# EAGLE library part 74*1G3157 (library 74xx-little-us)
Single-Pole, Double-Throw Analog Switch Source: http://focus.ti.com/lit/ds/symlink/sn74lvc1g3157.pdf
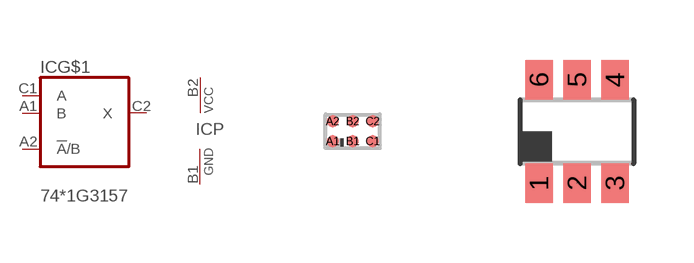
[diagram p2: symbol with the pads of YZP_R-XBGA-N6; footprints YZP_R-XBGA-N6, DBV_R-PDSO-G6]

Designator prefix IC; gates G$1=743157 P=PWRN-1

## 741G3157ZYPR  [YZP_R-XBGA-N6]
A1  G$1:B
A2  G$1:!A!/B  in
B1  P:GND  pwr
B2  P:VCC  pwr
C1  G$1:A
C2  G$1:X

## 741G3157DBVR  [DBV_R-PDSO-G6]
1  G$1:B
2  P:GND  pwr
3  G$1:A
4  G$1:X
5  P:VCC  pwr
6  G$1:!A!/B  in

## 741G3157DCKR  [DCK_R-PDSO-G6]
Pads as for DBV_R-PDSO-G6

## 741G3157DRLR  [DRL_R-PDSO-N6]
Pads as for DBV_R-PDSO-G6

## 741G3157YEPR  [YEP_R-XBGA-N6]
Pads as for YZP_R-XBGA-N6

## Footprint YZP_R-XBGA-N6 (pad centres in mm)
YZP (R-XBGA-N6) DIE-SIZE BALL GRID ARRAY NanoFree TM - WCSP (DSBGA) 0.23-mm Large Bump - YZP (Pb-free) Source: http://focus.ti.com/lit/ds/symlink/sn74lvc1g3157
smd 0.3 x 0.3: A1 -0.5,-0.25; A2 -0.5,0.25; B1 0,-0.25; B2 0,0.25; C1 0.5,-0.25; C2 0.5,0.25

## Footprint DBV_R-PDSO-G6 (pad centres in mm)
DBV (R-PDSO-G6) PLASTIC SMALL-OUTLINE PACKAGE SOT (SOT-23) - DBV Source: http://focus.ti.com/lit/ds/symlink/sn74lvc1g3157.
smd 0.69 x 0.99: 1 -0.95,-1.29; 2 0,-1.29; 3 0.95,-1.29; 4 0.95,1.3; 5 0,1.3; 6 -0.95,1.3

## Footprint DCK_R-PDSO-G6 (pad centres in mm)
DCK (R-PDSO-G6) PLASTIC SMALL-OUTLINE PACKAGE SOT (SC-70) - DCK Source: http://focus.ti.com/lit/ds/symlink/sn74lvc1g3157.
smd 0.4 x 0.7: 1 -0.65,-0.85; 2 0,-0.85; 3 0.65,-0.85; 4 0.65,0.85; 5 0,0.85; 6 -0.65,0.85

## Footprint DRL_R-PDSO-N6 (pad centres in mm)
DRL (R-PDSO-N6) PLASTIC SMALL OUTLINE SOT (SOT-553) - DRL Source: http://focus.ti.com/lit/ds/symlink/sn74lvc1g3157.pdf
smd 0.35 x 0.55: 1 -0.5,-0.675; 2 0,-0.675; 3 0.5,-0.675; 4 0.5,0.675; 5 0,0.675; 6 -0.5,0.675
